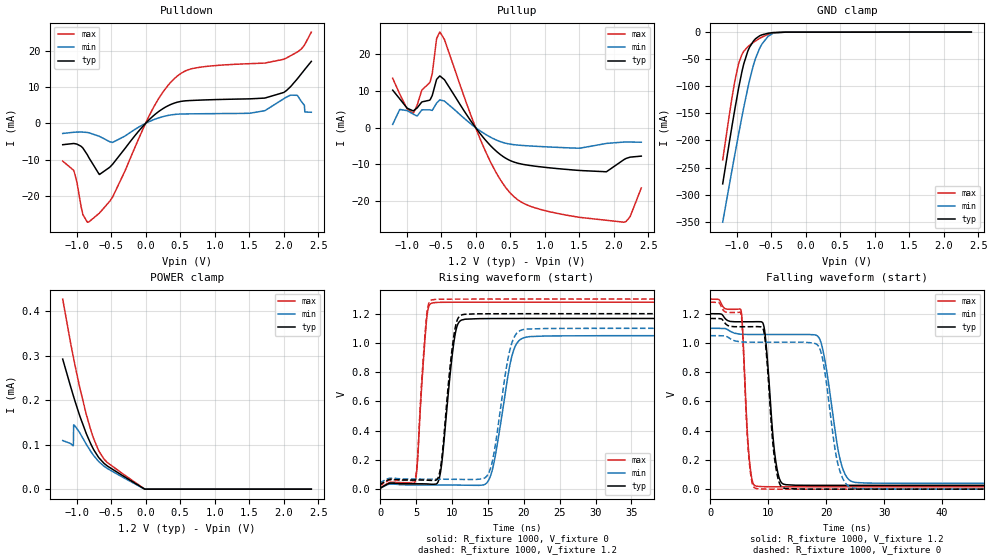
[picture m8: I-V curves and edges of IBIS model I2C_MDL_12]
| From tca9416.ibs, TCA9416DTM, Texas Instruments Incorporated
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[Model]   I2C_MDL_12
Model_type   I/O
Polarity   Non-Inverting
Enable   Active-High
Vinl = 0.36
Vinh = 0.84
Vmeas = 0.6
Vref = 0
Cref = 2pF
Rref = 100000
|   typ   min   max
C_comp   7.2608pF   6.6746pF   7.8469pF
[Voltage Range]   1.2   1.08   1.32
[Temperature Range]   27   125   -40
[Pullup Reference]   1.2   1.08   1.32
[Pulldown Reference]   0   -0   0
[Power Clamp Reference]   1.2   1.08   1.32
[GND Clamp Reference]   0   0   0
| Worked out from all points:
|   slope of the pulldown table from 0 to 0.18 V, typ, clamps not added: 57.9 ohm
|   slope of the pullup table from 0 to 0.18 V, typ, clamps not added: 43.1 ohm
|   GND clamp passes 1 mA (typ) near -0.48 V on its own axis
|   rising waveform, R_fixture 1000, V_fixture 0: 20-80 % time 1.38ns typ, 2.07ns min, 958ps max; typ from 0.001 V to 1.17 V
|   falling waveform, R_fixture 1000, V_fixture 1.2: 20-80 % time 1.38ns typ, 2.39ns min, 953ps max; typ from 1.2 V to 0.026 V
|   rising waveform, R_fixture 1000, V_fixture 1.2: 20-80 % time 1.34ns typ, 1.91ns min, 949ps max; typ from 0.026 V to 1.2 V
|   falling waveform, R_fixture 1000, V_fixture 0: 20-80 % time 1.34ns typ, 2.2ns min, 941ps max; typ from 1.17 V to 0.001 V
[Pulldown]
|I2C_MDL_12
|   Voltage   I(typ)   I(min)   I(max)
-1.2V     -5.87mA    -2.773mA   -10.37mA
-1.042V   -5.536mA   -2.455mA   -12.91mA
-908.4mV  -6.768mA   -2.407mA   -25.05mA
-822mV    -9.393mA   -2.574mA   -27.1mA
-667.2mV  -14.05mA   -3.588mA   -24.65mA
-476.4mV  -11.22mA   -5.236mA   -20.22mA
121.2mV   2.214mA    1.031mA    4.59mA
445.2mV   5.737mA    2.495mA    12.77mA
1.511V    6.733mA    2.785mA    16.41mA
2V        8.485mA    6.757mA    17.6mA
2.195V    12.17mA    7.694mA    19.58mA
2.4V      17.02mA    3.051mA    25.08mA
[GND Clamp]
|I2C_MDL_12
|   Voltage   I(typ)   I(min)   I(max)
-1.2V     -280.2mA   -350.9mA   -236mA
-1.063V   -171.7mA   -253.2mA   -119.3mA
-1.024V   -141.8mA   -225.4mA   -89.94mA
-966mV    -101mA     -185.9mA   -56.63mA
-894mV    -58.24mA   -138.4mA   -35.37mA
-807.6mV  -27.19mA   -86.99mA   -23.94mA
-732mV    -13.19mA   -51.35mA   -16.96mA
-667.2mV  -7.009mA   -30.48mA   -11.78mA
-541.2mV  -2.112mA   -7.698mA   -4.181mA
-454.8mV  -697.9uA   -1.65mA    -1.359mA
-296.4mV  -153.9uA   -154.6uA   -192.7uA
2.4V      0A         0A         0A
[Pullup]
|I2C_MDL_12
|   Voltage   I(typ)   I(min)   I(max)
-1.2V     10.19mA    879.4uA    13.43mA
-1.099V   7.846mA    4.906mA    9.17mA
-904.8mV  4.555mA    3.701mA    3.899mA
-660mV    7.56mA     4.812mA    12.44mA
-562.8mV  13.17mA    6.72mA     24.32mA
-516mV    14.06mA    7.535mA    26.02mA
207.6mV   -4.748mA   -2.539mA   -9.032mA
459.6mV   -8.602mA   -4.368mA   -16.9mA
711.6mV   -10.11mA   -4.918mA   -20.8mA
1.892V    -12.04mA   -4.33mA    -25.27mA
2.148V    -8.741mA   -3.949mA   -25.79mA
2.4V      -7.779mA   -3.992mA   -16.44mA
[POWER Clamp]
|I2C_MDL_12
|   Voltage   I(typ)   I(min)   I(max)
-1.2V     292.8uA    109.5uA    427.8uA
-1.049V   211.7uA    97.51uA    299.3uA
-1.045V   209.8uA    99.79uA    296.5uA
-1.042V   208uA      144.6uA    293.7uA
-948mV    162.7uA    125.3uA    225.2uA
-854.4mV  123.4uA    100uA      166uA
-764.4mV  92.74uA    78.41uA    119.5uA
-685.2mV  72.59uA    63.36uA    88.79uA
-606mV    58.77uA    52.21uA    68.59uA
-552mV    51.94uA    46.28uA    59.67uA
-4.8mV    0A         0A         0A
2.4V      0A         0A         0A
[Ramp]
|I2C_MDL_12
| variable   typ   min   max
dV/dt_r   0.70/1.37E-09   0.63/2.07E-09   0.77/9.59E-10
dV/dt_f   0.70/1.38E-09   0.64/2.38E-09   0.77/9.53E-10
R_load = 1000
[Rising Waveform]
|I2C_MDL_12
R_fixture =   1000
C_fixture =   0
L_fixture =   0
V_fixture =   0
V_fixture_min = 0
V_fixture_max = 0
|   Time   V(typ)   V(min)   V(max)
0s        637.3uV    824.7uV    478.3uV
4.889ns   37.21mV    29.03mV    57.62mV
6.473ns   36.3mV     28.97mV    1.167V
7.397ns   33.81mV    28.87mV    1.275V
10.48ns   1.07V      28.48mV    1.278V
11.84ns   1.163V     27.55mV    1.278V
15.23ns   1.167V     74.03mV    1.279V
18.44ns   1.167V     927.5mV    1.279V
20.86ns   1.167V     1.044V     1.279V
219.5ns   1.167V     1.05V      1.279V
[Falling Waveform]
|I2C_MDL_12
R_fixture =   1000
C_fixture =   0
L_fixture =   0
V_fixture =   1.2
V_fixture_min = 1.1
V_fixture_max = 1.3
|   Time   V(typ)   V(min)   V(max)
0s        1.2V       1.1V       1.3V
5.329ns   1.145V     1.06V      1.218V
6.693ns   1.145V     1.058V     223.5mV
8.057ns   1.145V     1.058V     20.36mV
11.49ns   145.1mV    1.058V     16.9mV
13.07ns   31mV       1.058V     16.83mV
18.88ns   26.57mV    1.026V     16.77mV
22.45ns   26.51mV    194.9mV    16.76mV
25.13ns   26.49mV    45.89mV    16.76mV
219.5ns   26.45mV    40.18mV    16.75mV
[Rising Waveform]
|I2C_MDL_12
R_fixture =   1000
C_fixture =   0
L_fixture =   0
V_fixture =   1.2
V_fixture_min = 1.1
V_fixture_max = 1.3
|   Time   V(typ)   V(min)   V(max)
0s        26.45mV    40.18mV    16.75mV
4.889ns   63.13mV    69.25mV    74.55mV
6.473ns   62.1mV     68.91mV    1.192V
7.573ns   60.21mV    68.62mV    1.297V
10.39ns   1.089V     67.75mV    1.3V
11.75ns   1.196V     66.7mV     1.3V
15.18ns   1.2V       118.6mV    1.3V
18.13ns   1.2V       965.5mV    1.3V
20.38ns   1.2V       1.095V     1.3V
219.5ns   1.2V       1.1V       1.3V
[Falling Waveform]
|I2C_MDL_12
R_fixture =   1000
C_fixture =   0
L_fixture =   0
V_fixture =   0
V_fixture_min = 0
V_fixture_max = 0
|   Time   V(typ)   V(min)   V(max)
0s        1.167V     1.05V      1.279V
5.329ns   1.111V     1.007V     1.196V
6.693ns   1.111V     1.005V     199.9mV
8.057ns   1.112V     1.005V     3.932mV
11.4ns    127.3mV    1.005V     631.9uV
13.03ns   4.952mV    1.006V     559.4uV
18.84ns   751.1uV    966.3mV    495.7uV
22.05ns   696.9uV    167.6mV    486.1uV
24.87ns   673.1uV    6.278mV    482.3uV
219.5ns   637.3uV    824.7uV    478.3uV
